FUNCTION_BLOCK FB_Visus IMPLEMENTS  I_Runtime

VAR
	ArrAxisPosition				AT%I* : ARRAY [1..5] OF LREAL;
	ArrAxisNotMoving			AT%I* : ARRAY [1..5] OF BOOL;	
END_VAR

METHOD Cyclic
//
END_METHOD

END_FUNCTION_BLOCK
